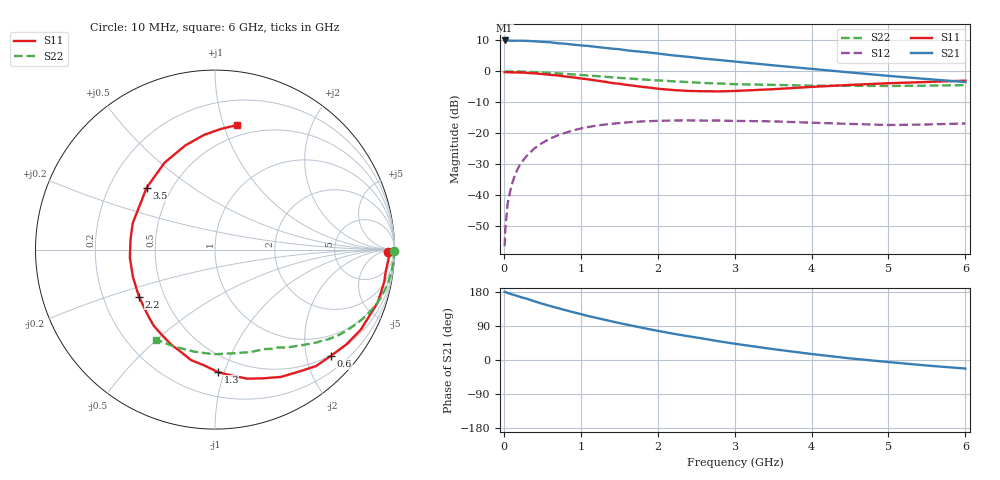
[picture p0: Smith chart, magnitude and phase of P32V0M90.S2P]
! SIEMENS Small Signal Semiconductors
! BFP181
! Si NPN RF Bipolar Junction Transistor in SOT143
! VCE = 2 V  IC = 0.9 mA
! Common Emitter S-Parameters:  March  1996
# GHz  S  MA  R  50
!  f  S11  S21  S12  S22
! GHz  MAG  ANG  MAG  ANG  MAG  ANG  MAG  ANG
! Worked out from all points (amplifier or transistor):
!   36 points, 10 MHz to 6 GHz, reference 50 ohm
!   highest |S21| = 10.0 dB at 10 MHz (marker M1)
!   |S21| within 3 dB of that: start of sweep to 1.546 GHz
!   unconditionally stable (mu >= 1): 3.163 GHz to end of sweep
!   at 250 MHz: K = 0.09, MSG = 19.3 dB, |S12| = -28.8 dB
!   at 1.4 GHz: K = 0.49, MSG = 12.1 dB, |S12| = -17.0 dB
!   at 6 GHz: K = 1.32, MAG = 3.3 dB, |S12| = -16.8 dB
!   S11 on the Smith chart (normalised r, x): 10 MHz: 48, -22; 600 MHz: 0.49, -2.49; 1.3 GHz: 0.37, -0.95; 2.2 GHz: 0.36, -0.25; 3.5 GHz: 0.36, +0.34; 6 GHz: 0.40, +1.11
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0.01  0.9658 -0.9  3.149 179.7  0.0015 82.3  0.9994 -0.3
0.02  0.9727 -1.5  3.142 179.4  0.0029 90.3  0.9918 -0.6
0.05  0.9673 -3.4  3.142 176.9  0.0074 90.7  0.997 -1.7
0.1  0.9591 -7.3  3.118 173.7  0.0145 83.9  0.9972 -3.4
0.15  0.9601 -10.7  3.111 170.5  0.0221 81.9  0.9941 -5.0
0.2  0.9551 -14.4  3.122 167.3  0.0297 80.9  0.9914 -6.8
0.3  0.9405 -21.6  3.1 161.6  0.0435 75.6  0.9839 -10.1
0.4  0.9266 -28.8  3.05 154.7  0.0572 71.2  0.9731 -13.3
0.6  0.8762 -42.5  2.947 142.8  0.0819 61.9  0.9444 -19.5
0.8  0.8237 -55.8  2.786 131.6  0.1017 53.6  0.9095 -25.0
1.1  0.7415 -75.9  2.567 115.8  0.1264 42.6  0.8552 -32.3
1.3  0.6825 -88.7  2.401 106.7  0.1376 35.7  0.8192 -36.7
1.5  0.6295 -102.3  2.273 97.5  0.1458 30.5  0.7827 -40.4
1.8  0.5602 -121.8  2.06 84.8  0.155 23.5  0.74 -45.3
2.2  0.4983 -148.3  1.807 69.5  0.1604 15.1  0.6902 -51.7
2.4  0.4819 -161.6  1.711 62.6  0.1611 11.5  0.6696 -54.6
2.8  0.4741 173.5  1.521 49.2  0.1604 5.9  0.636 -60.4
3.5  0.5139 137.8  1.249 28.7  0.1555 -1.2  0.6037 -71.1
4  0.56 120.1  1.094 15.8  0.1479 -4.0  0.5861 -80.4
4.5  0.6028 106.1  0.959 4.3  0.1415 -6.1  0.583 -90.7
5.5  0.6727 87.3  0.75 -14.6  0.1384 -2.2  0.586 -112.1
6  0.7055 79.8  0.671 -22.6  0.1438 -0.9  0.5991 -123.2
